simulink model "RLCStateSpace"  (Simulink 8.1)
settings: Solver=ode23t  StartTime=0.0  StopTime=100  RelTol=1e-3
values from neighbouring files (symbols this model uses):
  U = 5    [MotorDCParam.m]
undefined symbols (not defined in the file or in its folder): C, L, R

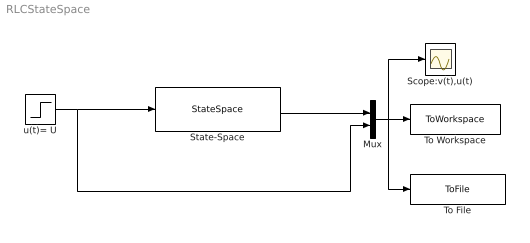
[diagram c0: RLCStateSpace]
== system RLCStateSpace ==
  Mux : Mux  Inputs=2
  Scope:v(t),u(t) : Scope
  State-Space : StateSpace  A=[0 1/C;-1/L -R/L]  B=[0; 1/L]  C=[1 0]  D=[0]
  To File : ToFile  Filename=RLCEstados.mat  SaveFormat=Timeseries
  To Workspace : ToWorkspace  VariableName=RLCEstados  SampleTime=-1
  u(t)= U : Step  Time=0  After=U  SampleTime=0
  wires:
  u(t)= U/1 -> Mux/2, State-Space/1
  State-Space/1 -> Mux/1
  Mux/1 -> To File/1, To Workspace/1, Scope:v(t),u(t)/1
